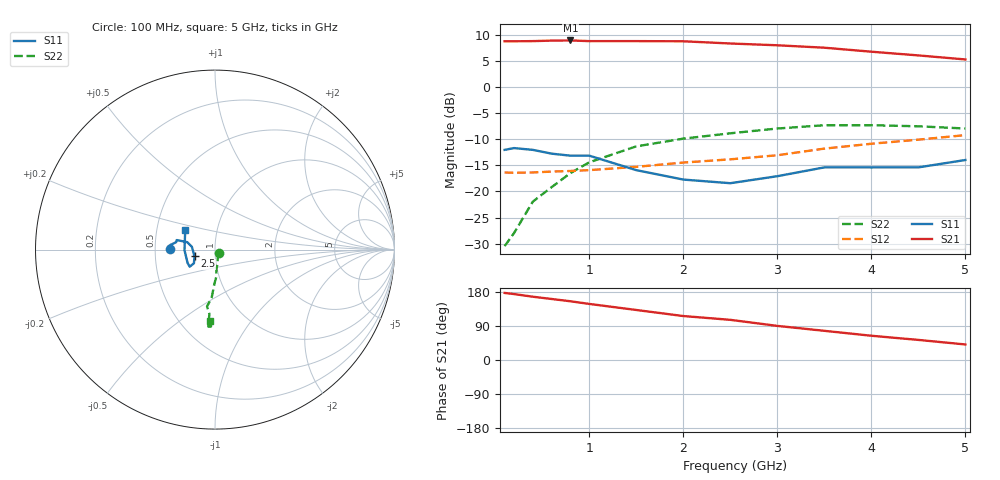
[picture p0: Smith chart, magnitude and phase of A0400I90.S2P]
!  MSA-0400 S PARAMETERS
!  Id = 90 mA  LAST UPDATED 07-22-92
# ghz s ma r 50
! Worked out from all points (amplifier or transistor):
!   14 points, 100 MHz to 5 GHz, reference 50 ohm
!   highest |S21| = 8.9 dB at 800 MHz (marker M1)
!   |S21| within 3 dB of that: start of sweep to 4.591 GHz
!   unconditionally stable (mu >= 1): start of sweep to 2.774 GHz
!   at 400 MHz: K = 1.32, MAG = 9.2 dB, |S12| = -16.4 dB
!   at 2 GHz: K = 1.09, MAG = 9.7 dB, |S12| = -14.5 dB
!   at 5 GHz: K = 0.88, MSG = 7.2 dB, |S12| = -9.2 dB
!   S11 on the Smith chart (normalised r, x): 100 MHz: 0.60, +0.01; 2.5 GHz: 0.79, -0.06; 5 GHz: 0.70, +0.16
0.1  0.25 179.0  2.73 177.0  0.152 2.0  0.03 -36.0
0.2  0.26 176.0  2.73 174.0  0.151 4.0  0.04 -67.0
0.4  0.25 174.0  2.74 167.0  0.152 4.0  0.08 -80.0
0.6  0.23 171.0  2.77 161.0  0.155 6.0  0.11 -86.0
0.8  0.22 169.0  2.78 155.0  0.157 9.0  0.15 -87.0
1  0.22 166.0  2.74 148.0  0.16 10.0  0.19 -91.0
1.5  0.16 165.0  2.74 132.0  0.172 16.0  0.27 -94.0
2  0.13 173.0  2.73 116.0  0.189 22.0  0.32 -98.0
2.5  0.12 -162.0  2.6 106.0  0.203 31.0  0.36 -95.0
3  0.14 -147.0  2.5 90.0  0.222 33.0  0.4 -95.0
3.5  0.17 -146.0  2.37 77.0  0.257 34.0  0.43 -95.0
4  0.17 -154.0  2.17 64.0  0.286 36.0  0.43 -93.0
4.5  0.17 -179.0  2 53.0  0.313 37.0  0.42 -93.0
5  0.2 146.0  1.83 41.0  0.346 36.0  0.4 -94.0
